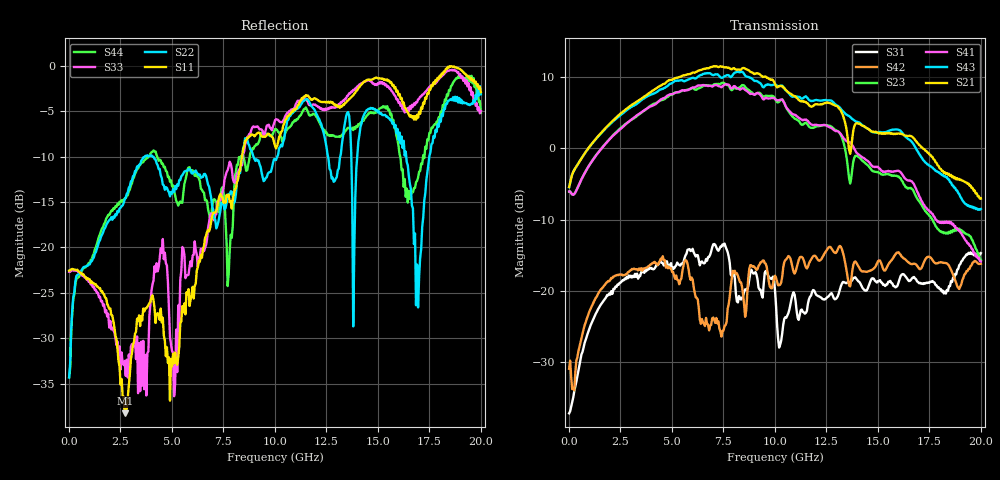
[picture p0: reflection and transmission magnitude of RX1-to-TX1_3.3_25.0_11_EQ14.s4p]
!Agilent Technologies,N5225A,MY51451112,A.09.50.13
!Agilent N5225A: A.09.50.13
!Date: Wednesday, January 31, 2018 11:06:00
!Correction: S11(Full 4 Port(1,2,3,4))
!S12(Full 4 Port(1,2,3,4))
!S13(Full 4 Port(1,2,3,4))
!S14(Full 4 Port(1,2,3,4))
!S21(Full 4 Port(1,2,3,4))
!S22(Full 4 Port(1,2,3,4))
!S23(Full 4 Port(1,2,3,4))
!S24(Full 4 Port(1,2,3,4))
!S31(Full 4 Port(1,2,3,4))
!S32(Full 4 Port(1,2,3,4))
!S33(Full 4 Port(1,2,3,4))
!S34(Full 4 Port(1,2,3,4))
!S41(Full 4 Port(1,2,3,4))
!S42(Full 4 Port(1,2,3,4))
!S43(Full 4 Port(1,2,3,4))
!S44(Full 4 Port(1,2,3,4))
!S4P File: Measurements: <S11,S12,S13,S14>,
!<S21,S22,S23,S24>,
!<S31,S32,S33,S34>,
!<S41,S42,S43,S44>:
# Hz S  RI  R 50
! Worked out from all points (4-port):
!   401 points, 10 MHz to 20 GHz, reference 50 ohm
!   strongest paths, dB at 10 MHz, 5.008 GHz, 10.01 GHz, 15 GHz, 20 GHz:
!     S21: -5.4, 9.6, 9.0, 2.2, -7.0
!     S43: -5.5, 9.1, 9.0, 2.2, -8.5
!     S41: -6.1, 7.6, 6.9, -2.6, -15.8
!     S23: -6.1, 7.5, 7.0, -3.3, -15.6
!     S42: -30.9, -17.3, -17.8, -15.8, -16.2
!     S31: -37.1, -17.1, -19.9, -18.6, -14.7
!   lowest |S11| = -38.3 dB at 2.709 GHz (marker M1), VSWR 1.02, Z = 49.1 - j0.815 ohm
!   |S11| at or under -10 dB: start of sweep to 8.405 GHz
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1e7  -0.0744 -0.00284  -0.000433 0.000603  0.014 0.000537  -0.000107 0.000362
     0.5359 0.0145  -0.0132 0.014  -0.4975 -0.00263  0.0265 0.0118
     0.0139 0.000555  -3.58e-05 0.000359  -0.0734 -0.00364  -0.000227 0.000535
     -0.4979 -0.00221  0.026 0.0118  0.5335 0.0133  -0.0128 0.0144
2.70865e9  -0.00894 -0.0083  0.0158 0.00345  0.0518 0.1105  0.0174 0.000778
           1.543 -1.017  0.1829 0.0164  -1.179 0.8708  0.1006 0.092
           0.0586 0.1074  0.0189 0.00396  0.00524 0.0231  0.021 0.000776
           -1.039 1.011  0.0878 0.0951  1.262 -1.289  0.1828 -0.0335
6.956525e9  -0.0346 0.1452  0.0132 -0.0152  0.1405 0.0578  0.0105 -0.0269
            -3.694 0.4252  0.1031 -0.133  2.653 -0.726  0.0239 0.0328
            0.1523 0.1333  0.0202 -0.0138  0.0253 0.1472  0.0234 -0.0305
            2.09 -1.716  0.0638 -0.00897  -2.659 1.91  0.0903 -0.1416
8.6057e9  0.00475 0.3888  4.16e-05 -0.00896  0.0613 0.043  -0.00573 -0.0181
          -0.6783 3.515  -0.118 0.3756  0.0263 -2.636  -0.0107 0.1291
          0.0902 0.0484  0.00901 -0.0169  0.0291 0.3826  -0.00948 -0.0334
          -1.128 -2.277  -0.0218 0.0693  1.128 2.982  0.2052 0.1669
1.045478e10  0.1403 0.4613  -0.0278 -0.0409  -0.000572 0.00824  -0.0545 -0.0122
             2.332 1.241  0.2694 0.2898  -2.03 -0.4785  0.0324 0.1841
             -0.0462 0.0442  -0.035 -0.0387  0.2255 0.4581  -0.0595 -0.0177
             -1.978 0.6316  0.0744 0.1412  2.625 -0.3022  0.3937 -0.1054
1.415292e10  0.6636 0.41  -0.0283 -0.00306  0.011 0.0978  -0.0127 0.0128
             0.2387 -1.451  0.4372 0.147  0.15 0.8318  0.1536 0.0408
             0.0238 0.1101  -0.0142 -0.00119  0.7533 0.2526  -0.022 0.0145
             0.7846 0.4058  0.1279 0.0582  -1.227 -0.8442  -0.1352 -0.4672
2e10  0.7121 0.0729  0.0231 0.0349  -0.0804 0.1578  0.0349 0.0208
      0.065 0.4403  0.6935 0.0744  -0.0322 -0.1623  0.1551 0.039
      -0.0785 0.1667  0.00622 0.0479  0.5631 -0.0227  0.0475 0.0206
      -0.16 -0.0214  0.1486 0.0454  0.3664 0.0823  -0.1513 -0.5311
